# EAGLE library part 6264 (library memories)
SRAM 8K x 8 bits
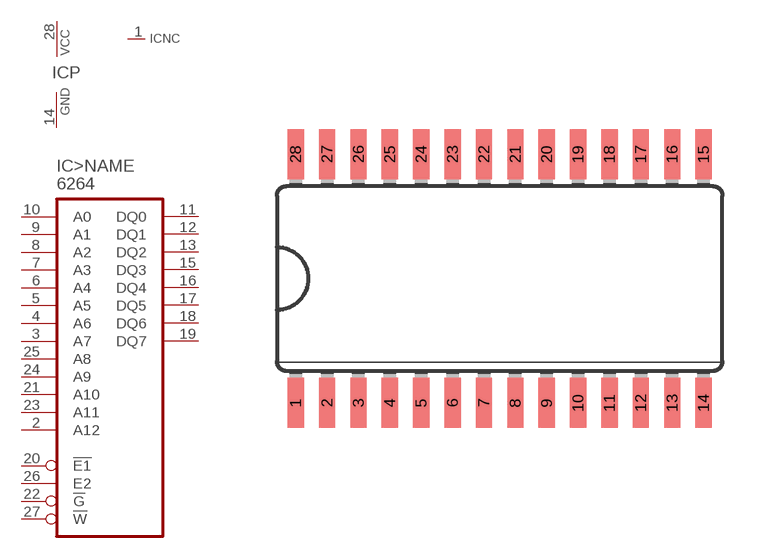
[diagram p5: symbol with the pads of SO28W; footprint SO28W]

Designator prefix IC; gates >NAME=RAM8KX8 P=PWRN NC=NC

## 6264  [SO28W]
1  NC:NC  nc
2  >NAME:A12  in
3  >NAME:A7  in
4  >NAME:A6  in
5  >NAME:A5  in
6  >NAME:A4  in
7  >NAME:A3  in
8  >NAME:A2  in
9  >NAME:A1  in
10  >NAME:A0  in
11  >NAME:DQ0
12  >NAME:DQ1
13  >NAME:DQ2
14  P:GND  pwr
15  >NAME:DQ3
16  >NAME:DQ4
17  >NAME:DQ5
18  >NAME:DQ6
19  >NAME:DQ7
20  >NAME:!E1  in
21  >NAME:A10  in
22  >NAME:!G  in
23  >NAME:A11  in
24  >NAME:A9  in
25  >NAME:A8  in
26  >NAME:E2  in
27  >NAME:!W  in
28  P:VCC  pwr

## Footprint SO28W (pad centres in mm)
Wide Small Outline package 300 mil
smd 0.66 x 2.032: 1 -8.255,-5.029; 2 -6.985,-5.029; 3 -5.715,-5.029; 4 -4.445,-5.029; 5 -3.175,-5.029; 6 -1.905,-5.029; 7 -0.635,-5.029; 8 0.635,-5.029; 9 1.905,-5.029; 10 3.175,-5.029; 11 4.445,-5.029; 12 5.715,-5.029; 13 6.985,-5.029; 14 8.255,-5.029; 15 8.255,5.029; 16 6.985,5.029; 17 5.715,5.029; 18 4.445,5.029; 19 3.175,5.029; 20 1.905,5.029; 21 0.635,5.029; 22 -0.635,5.029; 23 -1.905,5.029; 24 -3.175,5.029; 25 -4.445,5.029; 26 -5.715,5.029; 27 -6.985,5.029; 28 -8.255,5.029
